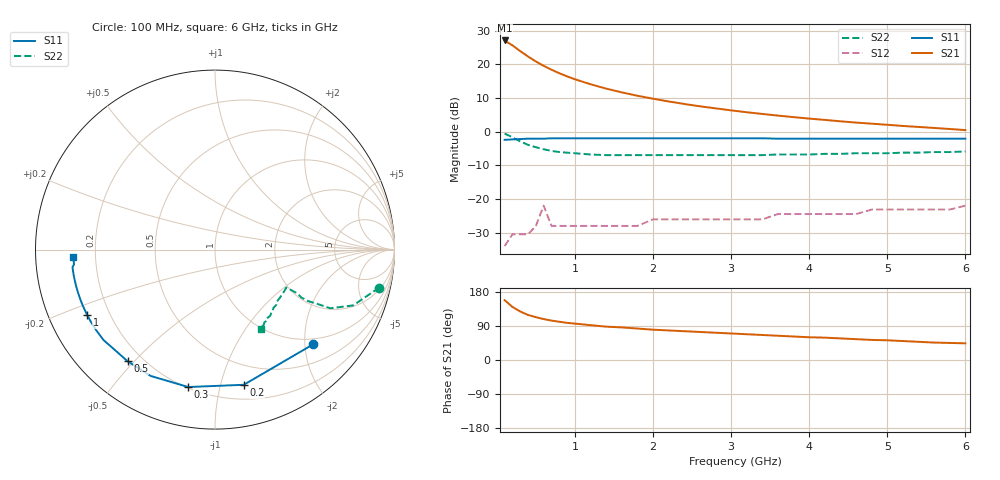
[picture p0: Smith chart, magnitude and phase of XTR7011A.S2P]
! HXTR-7011  Common Emitter
! Vce=10V  Ic=10ma
# ghz s ma r 50
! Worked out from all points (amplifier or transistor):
!   35 points, 100 MHz to 6 GHz, reference 50 ohm
!   highest |S21| = 27.1 dB at 100 MHz (marker M1)
!   |S21| within 3 dB of that: start of sweep to 290.8 MHz
!   unconditionally stable (mu >= 1): 2.531 GHz to end of sweep
!   at 600 MHz: K = 0.32, MSG = 20.8 dB, |S12| = -21.9 dB
!   at 2.6 GHz: K = 1.03, MAG = 15.7 dB, |S12| = -26.0 dB
!   at 6 GHz: K = 1.37, MAG = 7.6 dB, |S12| = -21.9 dB
!   S11 on the Smith chart (normalised r, x): 100 MHz: 0.87, -2.18; 200 MHz: 0.32, -1.18; 300 MHz: 0.21, -0.80; 500 MHz: 0.14, -0.48; 1 GHz: 0.12, -0.24; 6 GHz: 0.12, -0.03
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0.1  0.76 -44.0  22.72 158.0  0.02 70.0  0.94 -13.0
0.2  0.77 -78.0  19.2 140.0  0.03 54.0  0.83 -22.0
0.3  0.78 -101.0  15.8 128.0  0.03 44.0  0.72 -27.0
0.4  0.79 -117.0  13.11 119.0  0.03 37.0  0.64 -28.0
0.5  0.79 -128.0  11.08 113.0  0.04 33.0  0.59 -29.0
0.6  0.79 -135.0  9.54 108.0  0.08 30.0  0.55 -29.0
0.7  0.8 -141.0  8.35 104.0  0.04 29.0  0.52 -28.0
0.8  0.8 -146.0  7.41 101.0  0.04 27.0  0.5 -28.0
0.9  0.8 -150.0  6.65 98.0  0.04 27.0  0.49 -28.0
1  0.8 -153.0  6.03 96.0  0.04 26.0  0.48 -28.0
1.2  0.8 -157.0  5.08 92.0  0.04 26.0  0.46 -28.0
1.4  0.8 -160.0  4.38 88.0  0.04 27.0  0.45 -28.0
1.6  0.8 -163.0  3.85 86.0  0.04 27.0  0.45 -29.0
1.8  0.8 -165.0  3.43 83.0  0.04 28.0  0.45 -29.0
2  0.8 -167.0  3.1 80.0  0.05 29.0  0.45 -31.0
2.2  0.8 -168.0  2.82 78.0  0.05 30.0  0.45 -32.0
2.6  0.8 -170.0  2.39 74.0  0.05 32.0  0.45 -34.0
3.2  0.8 -172.0  1.95 68.0  0.05 34.0  0.45 -39.0
3.6  0.79 -174.0  1.74 64.0  0.06 35.0  0.46 -42.0
4.2  0.79 -175.0  1.5 59.0  0.06 37.0  0.47 -47.0
5.2  0.79 -176.0  1.22 50.0  0.07 39.0  0.49 -54.0
6  0.79 -177.0  1.06 44.0  0.08 39.0  0.51 -60.0
